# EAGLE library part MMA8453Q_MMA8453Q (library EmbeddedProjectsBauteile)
3-Axis, 8-bit/12-bit Digital Accelerometer
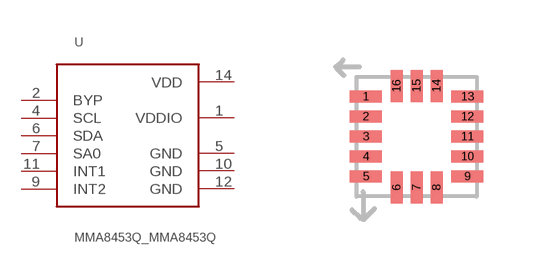
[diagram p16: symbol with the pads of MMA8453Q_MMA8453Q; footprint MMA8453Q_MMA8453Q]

Designator prefix -

## MMA8453Q_MMA8453Q (EP: 400299)  [MMA8453Q_MMA8453Q]
1  VDDIO  pwr
2  BYP
4  SCL
5  GND  sup
6  SDA
7  SA0
9  INT2
10  GND  sup
11  INT1
12  GND  sup
14  VDD  pwr

## Footprint MMA8453Q_MMA8453Q (pad centres in mm)
smd 0.8 x 0.3: 1 -1.27,1; 2 -1.27,0.5; 3 -1.27,0; 4 -1.27,-0.5; 5 -1.27,-1; 9 1.27,-1; 10 1.27,-0.5; 11 1.27,0; 12 1.27,0.5; 13 1.27,1
smd 0.3 x 0.8: 6 -0.5,-1.27; 7 0,-1.27; 8 0.5,-1.27; 14 0.5,1.27; 15 0,1.27; 16 -0.5,1.27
